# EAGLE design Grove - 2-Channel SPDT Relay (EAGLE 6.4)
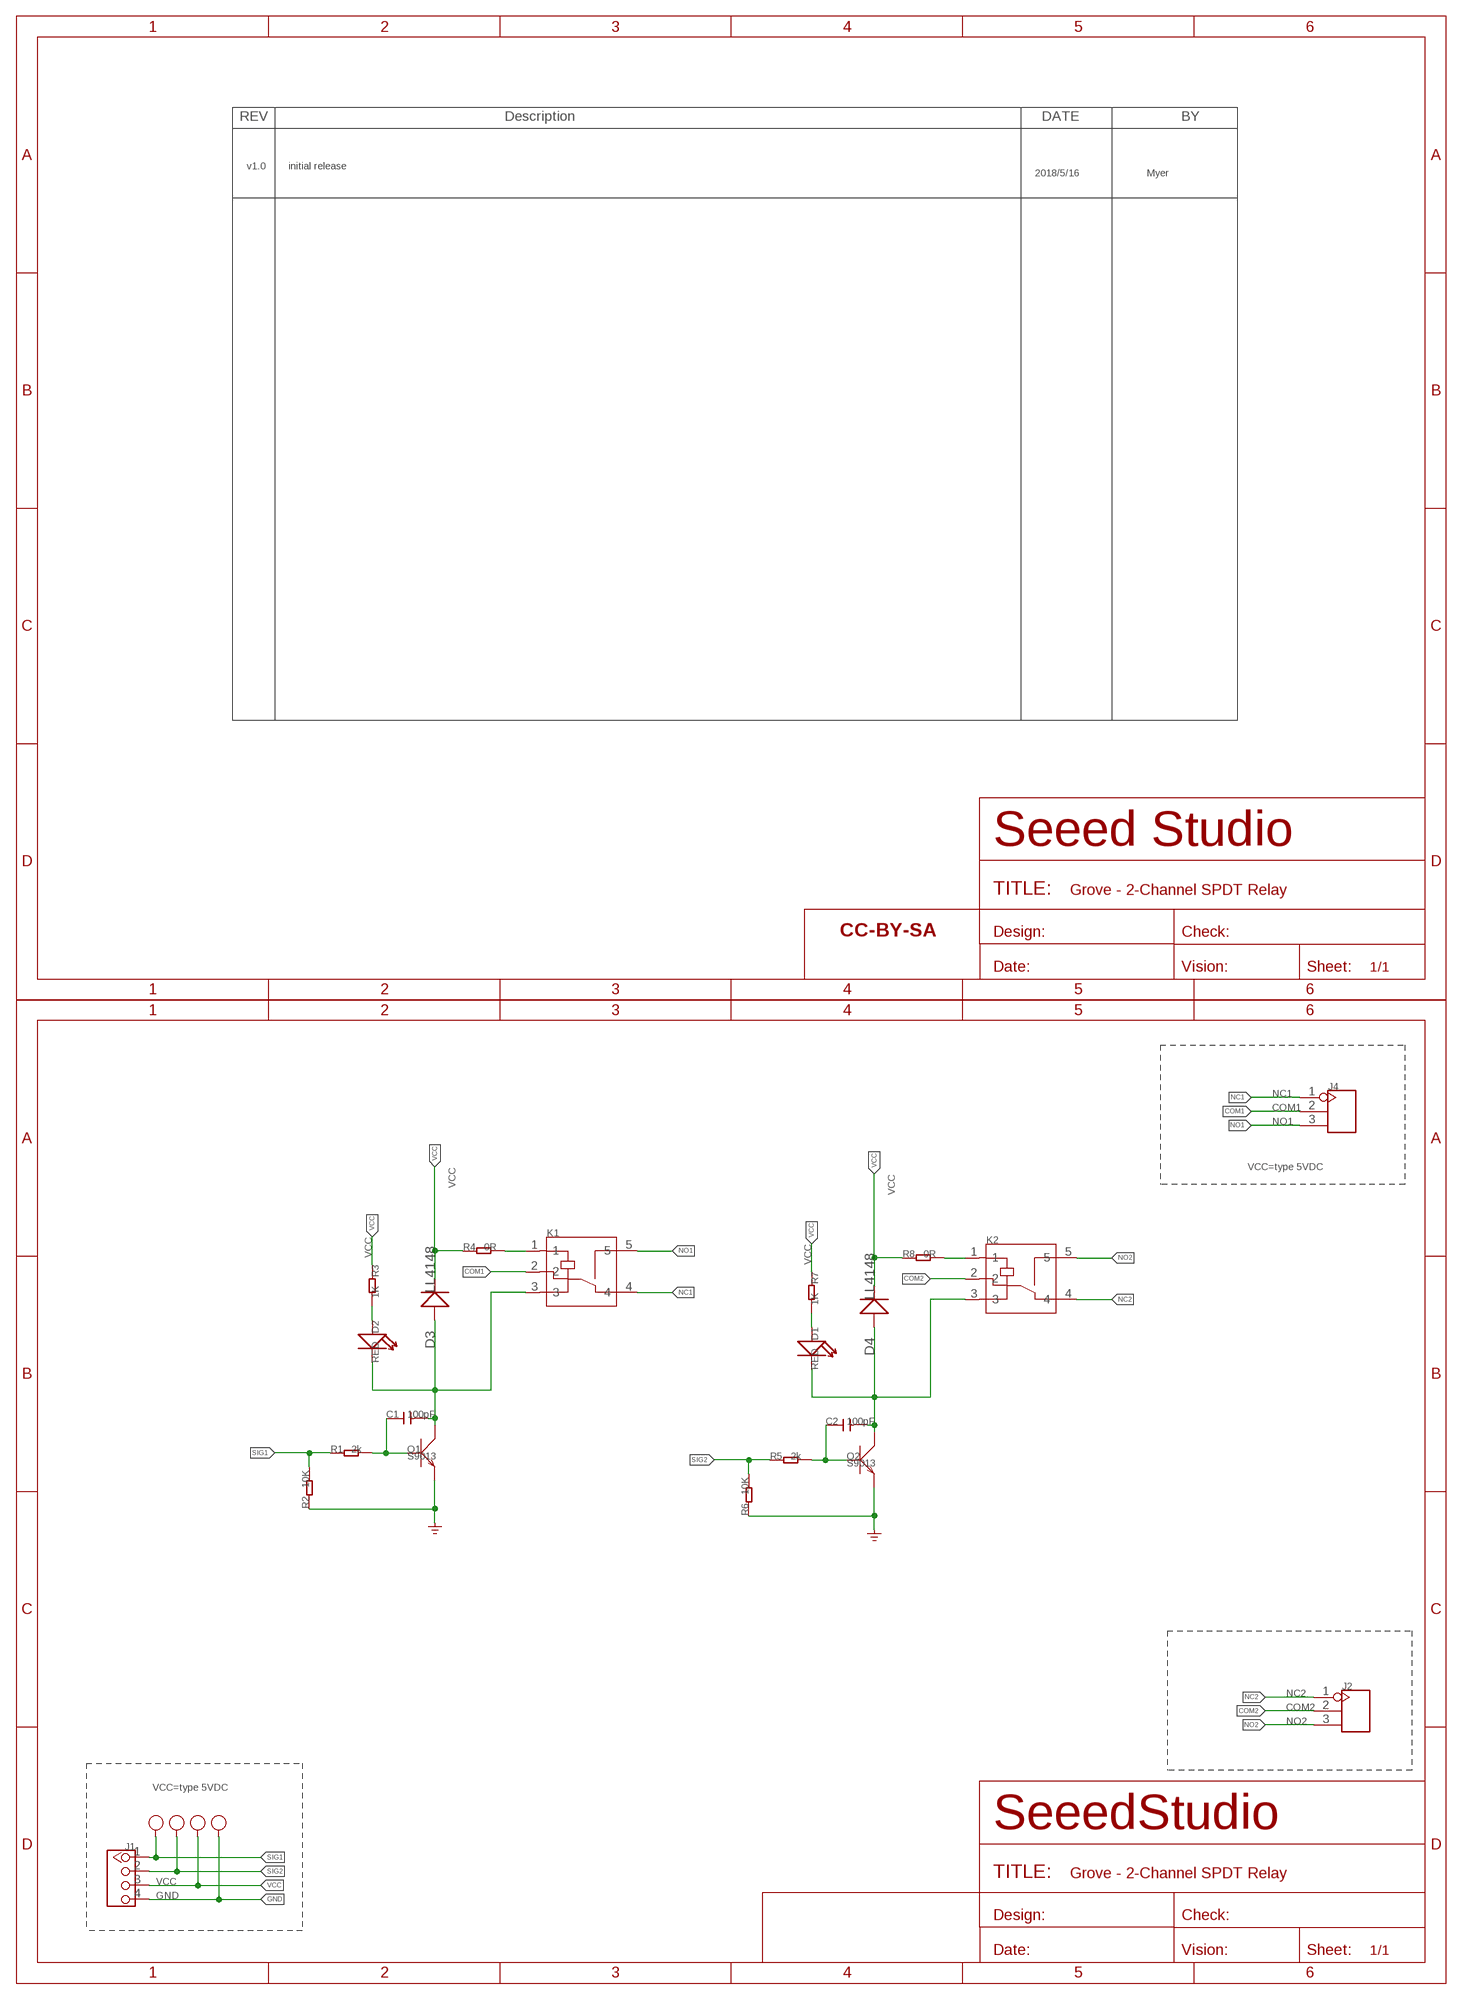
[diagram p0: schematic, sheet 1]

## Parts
C1  100pF  C-0603  [C0603]
C2  100pF  C-0603  [C0603]
D1  RED  LED'0603'  [LED-0603]
D2  RED  LED'0603'  [LED-0603]
D3  LL4148  D'1N4148-SMD'  [DO-35-SMD]
D4  LL4148  D'1N4148-SMD'  [DO-35-SMD]
FR2  SEEEDSTUDIO-OPEN-SCH-FRAME  [SEEEDSTUDIO-PCB-FRAME]
GND  TEST-POINT'4545'  [TP-D45MIL]
GND1  TEST-POINT'4545'  [TP-D45MIL]
GND2  TEST-POINT'4545'  [TP-D45MIL]
GND3  TEST-POINT'4545'  [TP-D45MIL]
J1  TWIG-4P-2.0-2.0  [4P-2.0]
J2  SCREW-TERMINAL-3P'5.08'  [3P-5.08]
J4  SCREW-TERMINAL-3P'5.08'  [3P-5.08]
K1  RELAY-SRD  [REY5-6-19.1X15.5X15.3MM]
K2  RELAY-SRD  [REY5-6-19.1X15.5X15.3MM]
Q1  S9013  TRANSISTOR-NPN-SOT23  [SOT23]
Q2  S9013  TRANSISTOR-NPN-SOT23  [SOT23]
R1  2k  R-0603  [R0603]
R2  10K  R-0603  [R0603]
R3  1K  R-0603  [R0603]
R4  0R  R-0603  [R0603]
R5  2k  R-0603  [R0603]
R6  10K  R-0603  [R0603]
R7  1K  R-0603  [R0603]
R8  0R  R-0603  [R0603]

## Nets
COM1: J4.2 K1.2
COM2: J2.2 K2.2
GND: GND3.T J1.4 Q1.2(E) Q2.2(E) R2.1 R6.1
N$1: C1.1 Q1.1(B) R1.2
N$2: D2.+ R3.2
N$3: K1.1 R4.2
N$4: C2.1 Q2.1(B) R5.2
N$5: D1.+ R7.2
N$6: C1.2 D2.- D3.A(+) K1.3 Q1.3(C)
N$7: C2.2 D1.- D4.A(+) K2.3 Q2.3(C)
N$8: K2.1 R8.2
NC1: J4.1 K1.4
NC2: J2.1 K2.4
NO1: J4.3 K1.5
NO2: J2.3 K2.5
SIG1: GND.T J1.1 R1.1 R2.2
SIG2: GND1.T J1.2 R5.1 R6.2
VCC: D3.C(-) D4.C(-) GND2.T J1.3 R3.1 R4.1 R7.1 R8.1

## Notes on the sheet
- v1.0 | initial release
- 2018/5/16 | Myer
- VCC=type 5VDC
- VCC=type 5VDC

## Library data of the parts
C1 C2 = Discrete:C*: Ceramic Capacitors
D1 D2 = Discrete:LED*
D3 D4 = Discrete:D*
FR2 = moudle-new:SEEEDSTUDIO-OPEN-SCH-FRAME
GND GND1-GND3 = Discrete-new:TEST-POINT; PARTNO: DNP
J1 = Connector:TWIG-4P-2.0
J2 J4 = Connector:SCREW-TERMINAL-3P
K1 K2 = Discrete-new:RELAY-SRD
Q1 Q2 = Discrete:TRANSISTOR-NPN*: NPN audion
R1-R8 = Discrete:R*

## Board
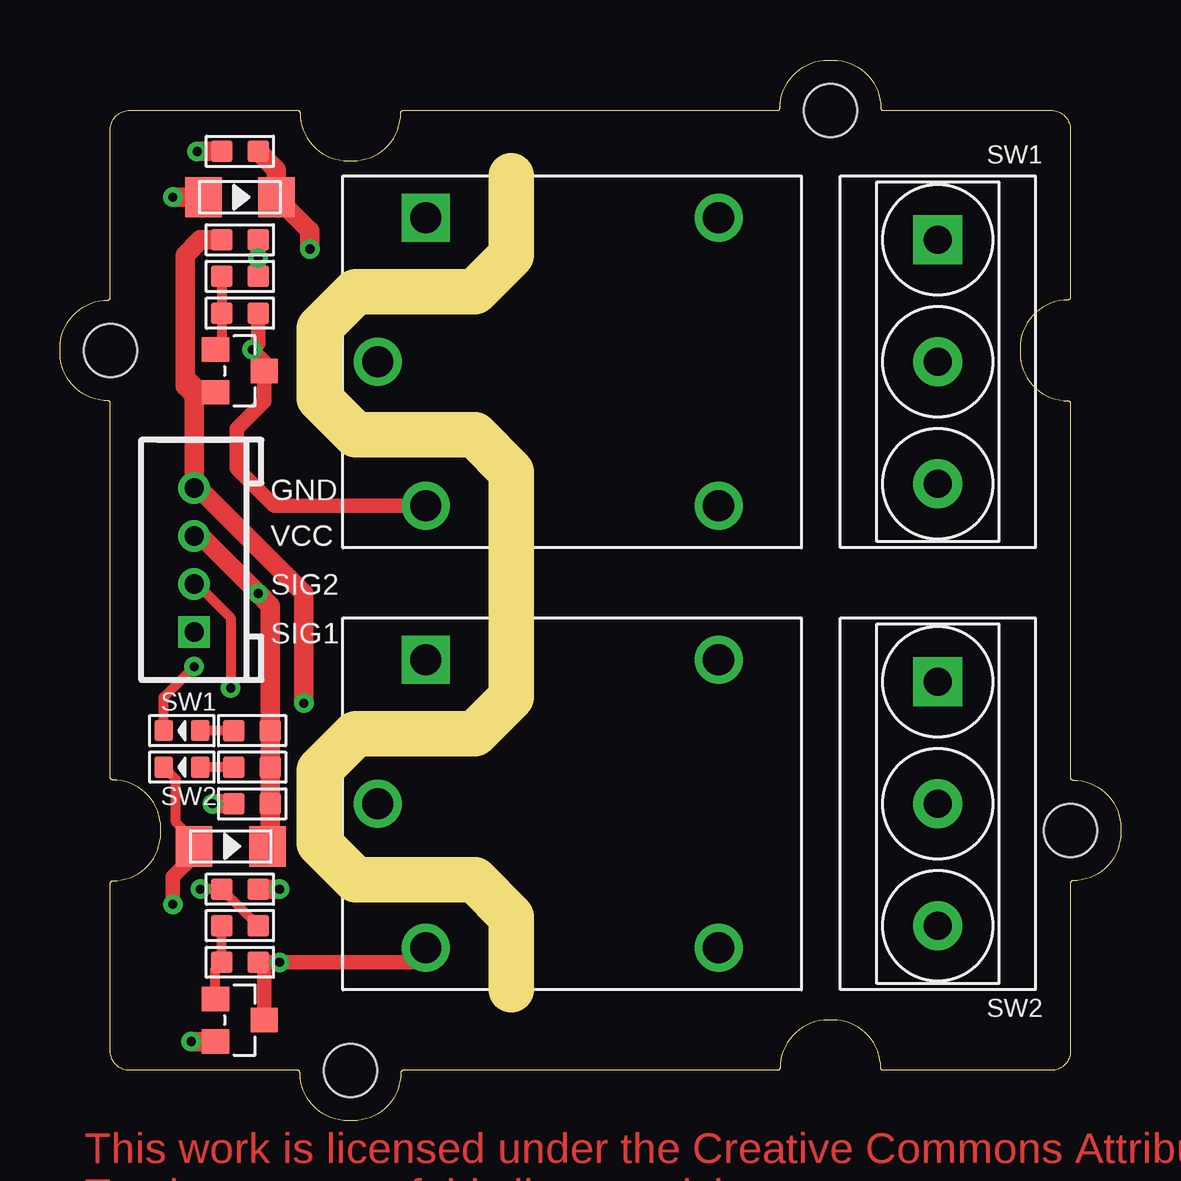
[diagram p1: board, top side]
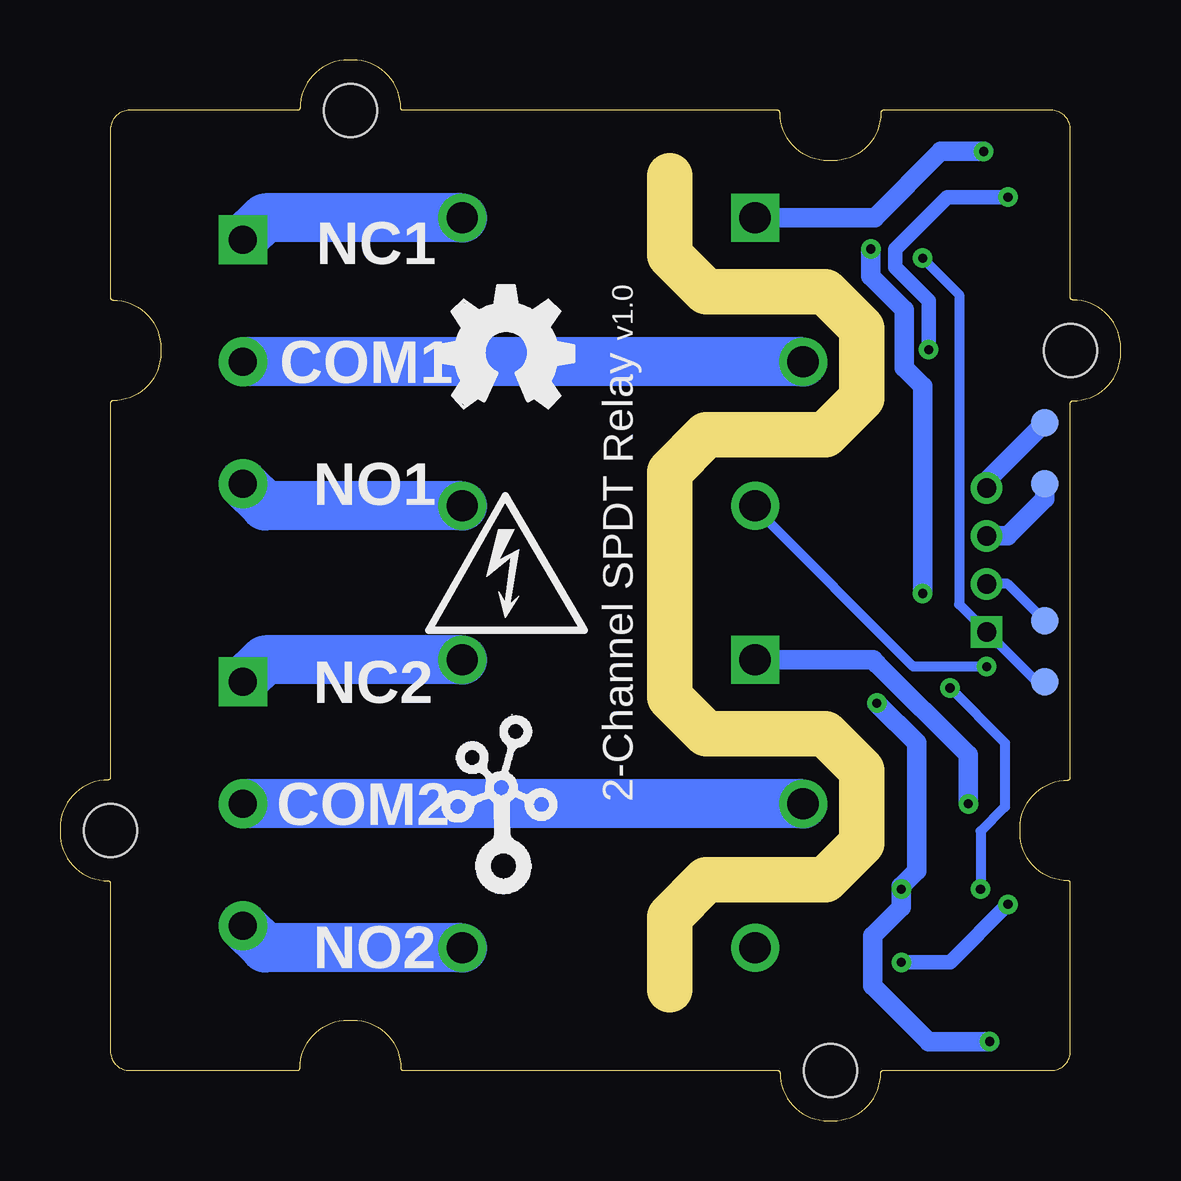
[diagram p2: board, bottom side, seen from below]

Size 44.2 x 44.2 mm. Coordinates in mm from the lower left corner, seen from the top.
Outline: 18.8,39.37 18.8,36.07 17.27,34.55 12.32,34.55 10.8,33.02 10.8,30.1 12.32,28.58 17.27,28.58 18.8,27.05 18.8,17.66 17.27,16.13 12.32,16.13 10.8,14.61 10.8,11.56 12.32,10.04 17.27,10.04 18.8,8.51 18.8,5.46
Copper layers (1*16): Top 0.035mm / dielectric 1.5mm / Bottom 0.035mm
Design rules "SeeedStudio_rule_no_angle_090911 *": minimum track width 6mil, minimum drill 12mil, track to track 6mil, track to pad 6mil, pad to pad 6mil, via to via 6mil, smd to smd 0mil, copper to edge 10mil, drill to drill 10mil, minimum pad ring 10mil, minimum via ring 6mil, stop-mask expansion 2mil, vias tented up to drill 25mil, thermal gap 10mil

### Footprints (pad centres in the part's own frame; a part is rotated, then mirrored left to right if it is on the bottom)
C0603 = smd 0.889 x 0.889: 1 -0.762,0; 2 0.762,0
LED-0603 = smd 0.762 x 0.889: + -0.762,0; - 0.762,0
DO-35-SMD = smd 1.524 x 1.676: A -1.524,0; C 1.524,0
TP-D45MIL = smd 1.143 x 1.143: T 0,0
4P-2.0 = drill 0.8 pad 1.27 square: 1 -3,0 | drill 0.8 pad 1.27: 2 -1,0; 3 1,0; 4 3,0
3P-5.08 = drill 1.168 pad 2.032 square: 1 0,5.08 | drill 1.168 pad 2.032: 2 0,0; 3 0,-5.08
REY5-6-19.1X15.5X15.3MM = drill 1.3 pad 2 square: 1 -6.1,6 | drill 1.3 pad 2: 2 -8.1,0; 3 -6.1,-6; 4 6.1,6; 5 6.1,-6
SOT23 = smd 1.016 x 1.143: 1 -0.889,-1.016; 2 0.889,-1.016; 3 0,1.016
R0603 = smd 0.889 x 0.889: 1 -0.762,0; 2 0.762,0
2X2U-DIM-W/-DRILL = hole 2.2: 10,20; -20,10; -10,-20; 20,-10

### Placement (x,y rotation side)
C1  7.5,33.66 0 top
C2  7.5,6.61 0 top
D1  5.08,14.73 180 top
D2  5.08,16.26 180 top
D3  7.5,38.48 0 top
D4  7.11,11.43 0 top
FR2  not placed on the board
GND  3.18,18.29 90 bottom
GND1  3.18,20.83 0 bottom
GND2  3.18,26.55 90 bottom
GND3  3.18,29.09 0 bottom
J1  5.59,23.37 90 top
J2  36.58,13.21 0 top
J4  36.58,31.62 0 top
K1  21.34,31.62 0 top
K2  21.34,13.21 0 top
Q1  7.5,31.24 270 top
Q2  7.5,4.19 270 top
R1  7.5,35.18 180 top
R2  7.5,36.7 0 top
R3  8,16.26 180 top
R4  7.5,40.39 180 top
R5  7.5,8.13 180 top
R6  7.5,9.65 180 top
R7  8,14.73 180 top
R8  8,13.21 180 top
U$3  [2X2U-DIM-W/-DRILL]  22.1,22.1 0 top
U$4  [OSHW_FILLX200_NOTEXT]  28.45,29.72 0 bottom
U$5  [TWIGLOGO]  25.78,10.42 0 bottom

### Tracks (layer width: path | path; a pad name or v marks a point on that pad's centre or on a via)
COM1
  Bottom 2.032: K1.2 J4.2
COM2
  Bottom 2.032: K2.2 J2.2
GND  (via drill 0.38 pad 0.81)
  Top 0.813: R2.1 5.84,36.7 5.21,36.07 5.21,30.99 | 5.21,30.99 5.21,30.74 | 5.21,30.74 5.21,30.61 5.46,30.36 Q1.2 | 5.21,30.99 5.72,30.48 | 5.21,30.74 5.59,30.36 J1.4 5.77,26.37 9.4,22.74 9.53,22.61 10.16,21.97 v10.16,17.4 | Q2.2 v5.46,3.3 | R6.1 v9.15,9.65
  Bottom 0.813: J1.4 5.59,26.67 GND3.T | v5.46,3.3 8,3.3 10.34,5.64 10.34,7.7 9.15,8.89 v9.15,9.65 9.15,9.78 8.51,10.42 8.51,15.75 v10.16,17.4
N$1
  Top 0.406: R1.2 C1.1 6.73,32.39 Q1.1
N$2
  Top 0.406: R3.2 D2.+
N$3  (via drill 0.38 pad 0.81)
  Top 0.813: R4.2 v5.72,40.39
  Bottom 0.813: K1.1 10.26,37.62 7.5,40.39 v5.72,40.39
N$4
  Top 0.406: Q2.1 6.48,6.35 C2.1 R5.2
N$5
  Top 0.406: R7.2 D1.+
N$6  (via drill 0.38 pad 0.81)
  Top 0.406: D2.- 4.32,17.66 v5.59,18.93
  Top 0.61: K1.3 8.92,25.62 7.37,27.18 7.37,28.83 8.51,29.97 Q1.3 8.51,31.62 v8,32.13 8.26,32.39 C1.2
  Top 0.813: D3.A v4.7,38.48
  Bottom 0.406: K1.3 15.24,25.53 8.64,18.93 v5.59,18.93
  Bottom 0.61: v4.7,38.48 7.24,38.48 9.4,36.32 9.4,35.56 8,34.16 v8,32.13
N$7  (via drill 0.38 pad 0.81)
  Top 0.406: D4.A 5.59,11.69 4.83,12.45 4.83,14.23 D1.-
  Top 0.61: Q2.3 8.51,6.35 C2.2 v9.15,6.61 14.63,6.61 K2.3 | v4.7,9.02 4.7,10.16 5.59,11.05 D4.A
  Bottom 0.61: v9.15,6.61 7.11,6.61 v4.7,9.02
N$8  (via drill 0.38 pad 0.81)
  Top 0.813: R8.2 v6.35,13.21
  Bottom 0.813: K2.1 10.32,19.21 10.29,19.18 10.16,19.05 6.35,15.24 v6.35,13.21
NC1
  Bottom 2.032: K1.4 35.66,37.62 J4.1
NC2
  Bottom 2.032: K2.4 35.66,19.21 J2.1
NO1
  Bottom 2.032: K1.5 35.66,25.62 J4.3
NO2
  Bottom 2.032: K2.5 35.66,7.21 J2.3
SIG1  (via drill 0.38 pad 0.81)
  Top 0.406: R2.2 v8.26,35.94 R1.1
  Bottom 0.406: GND.T 3.51,18.29 J1.1 6.73,21.51 6.73,34.42 v8.26,35.94
SIG2  (via drill 0.38 pad 0.81)
  Top 0.406: J1.2 5.7,22.37 7.11,20.96 v7.11,18.04 | R5.1 R6.2 v5.84,9.65
  Bottom 0.406: GND1.T 4.72,22.37 J1.2 | v7.11,18.04 4.83,15.75 4.83,13.08 5.84,12.07 v5.84,9.65
VCC  (via drill 0.38 pad 0.81)
  Top 0.813: R4.1 9.02,39.63 D3.C 10.42,37.09 v10.42,36.32 | J1.3 5.86,24.37 v8.26,21.97 8.77,21.46 R3.1 R7.1 R8.1 8.77,11.56 D4.C
  Bottom 0.813: J1.3 4.72,24.37 3.18,25.91 GND2.T | v8.26,21.97 8.26,30.61 9.02,31.37 9.02,33.78 10.42,35.18 v10.42,36.32

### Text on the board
tPlace: SW1 | GND | VCC | SIG2 | SIG1 | SW1 | SW2 | SW2
bPlace: NC1 | v1.0 | 2-Channel SPDT Relay | COM1 | NO1 | NC2 | COM2 | NO2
